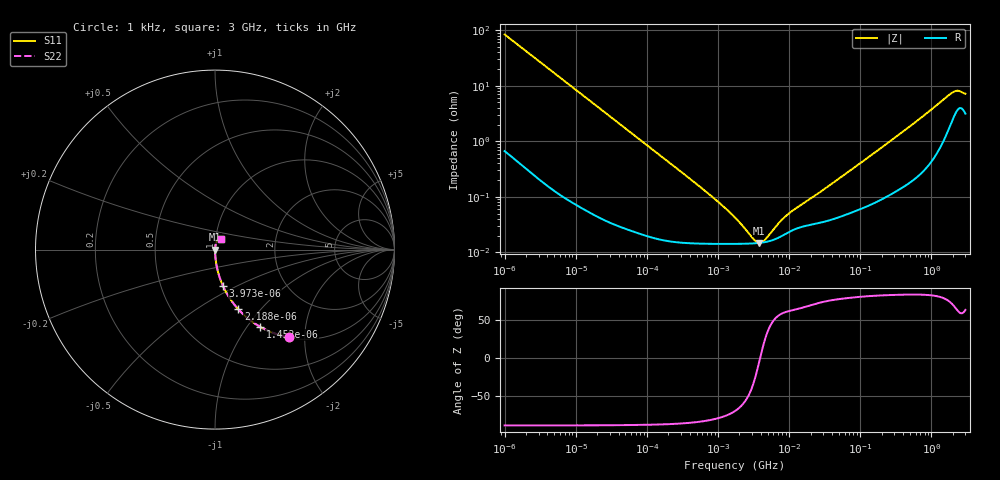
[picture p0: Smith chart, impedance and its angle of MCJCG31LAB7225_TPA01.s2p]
! MCJCG31LAB7225_TPA01  S-PARAMETER MODEL  ( Standard Model )
! Model Generated by TAIYO YUDEN Corporation (http://www.ty-top.com)
! Version 1.0
! TAIYO YUDEN Control No. 220601
! Copyright(c) 2015 TAIYO YUDEN CO.,LTD. All Rights Reserved.
! Product Description (link to TY-COMPAS)
! https://ds.yuden.co.jp/TYCOMPAS/or/detail?pn=MCJCG31LAB7225KTPA01&u=M
! Products Name : Multilayer Ceramic Capacitors
! Characteristics :
!  Capacitance : 2.2 [uF] , Rated Voltage : 35 [V] , TCC : X7R
!  Case Size : 3.2 x 1.6 / 0.126 x 0.063 [mm/inch] , Thickness : 1.6 / 0.063 [mm/inch]
!  (Conditions: Temperature = 25 [degC] , DC Bias Voltage = 0 [V])
! External Node Assignments :
!  1  o---| |---o  2
! GND o---------o GND
! Frequency Range : 1kHz  -  3GHz  [ 401 STEP ]
# MHZ S RI R 50
! Freq[MHz].  S11 Real  S11 Imag  S21 Real  S21 Imag  S12 Real  S12 Imag  S22 Real  S22 Imag
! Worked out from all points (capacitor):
!   401 points, 1 kHz to 3 GHz, reference 50 ohm
!   read as one part in series: C = 1.9 uF near 1.077 kHz
!   lowest |Z| = 14.8 mohm at 3.79 MHz (marker M1)
!   series resonance near 3.904 MHz, so ESL is about 870 pH
!   S11 on the Smith chart (normalised r, x): 1 kHz: 1.01, -1.67; 1.452 kHz: 1.01, -1.15; 2.188 kHz: 1.01, -0.77; 3.973 kHz: 1.00, -0.42; 3 GHz: 1.06, +0.13
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0.001  0.4119 -0.4882  0.5881 0.4882  0.5881 0.4882  0.4119 -0.4882
0.001452  0.2514 -0.4299  0.7486 0.4299  0.7486 0.4299  0.2514 -0.4299
0.002188  0.1301 -0.3327  0.8699 0.3327  0.8699 0.3327  0.1301 -0.3327
0.003973  0.0443 -0.2021  0.9557 0.2021  0.9557 0.2021  0.0443 -0.2021
0.006696  0.0165 -0.1237  0.9835 0.1237  0.9835 0.1237  0.0165 -0.1237
0.01216  0.00542 -0.0691  0.9946 0.0691  0.9946 0.0691  0.00542 -0.0691
0.033275  0.000974 -0.0255  0.999 0.0255  0.999 0.0255  0.000974 -0.0255
0.147855  0.000205 -0.00578  0.9998 0.00578  0.9998 0.00578  0.000205 -0.00578
0.791611  0.000143 -0.00104  0.9999 0.00104  0.9999 0.00104  0.000143 -0.00104
1.732051  0.000142 -0.000399  0.9999 0.000399  0.9999 0.000399  0.000142 -0.000399
3.14518  0.000145 -9.67e-05  0.9999 9.67e-05  0.9999 9.67e-05  0.000145 -9.67e-05
3.789741  0.000148 -1.32e-05  0.9999 1.32e-05  0.9999 1.32e-05  0.000148 -1.32e-05
4.083148  0.000149 2e-05  0.9999 -2e-05  0.9999 -2e-05  0.000149 2e-05
4.566395  0.000153 7.03e-05  0.9998 -7.03e-05  0.9998 -7.03e-05  0.000153 7.03e-05
7.143107  0.000185 0.000282  0.9998 -0.000282  0.9998 -0.000282  0.000185 0.000282
9.273352  0.000221 0.000411  0.9998 -0.000411  0.9998 -0.000411  0.000221 0.000411
21.06097  0.000318 0.000916  0.9997 -0.000916  0.9997 -0.000916  0.000318 0.000916
256.0921  0.00116 0.0097  0.9988 -0.0097  0.9988 -0.0097  0.00116 0.0097
783.755  0.00378 0.0287  0.9962 -0.0287  0.9962 -0.0287  0.00378 0.0287
1917.819  0.0261 0.067  0.9739 -0.067  0.9739 -0.067  0.0261 0.067
2310.849  0.0396 0.0674  0.9604 -0.0674  0.9604 -0.0674  0.0396 0.0674
3000  0.0342 0.0603  0.9658 -0.0603  0.9658 -0.0603  0.0342 0.0603
